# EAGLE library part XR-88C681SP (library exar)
DUAL UART full duplex
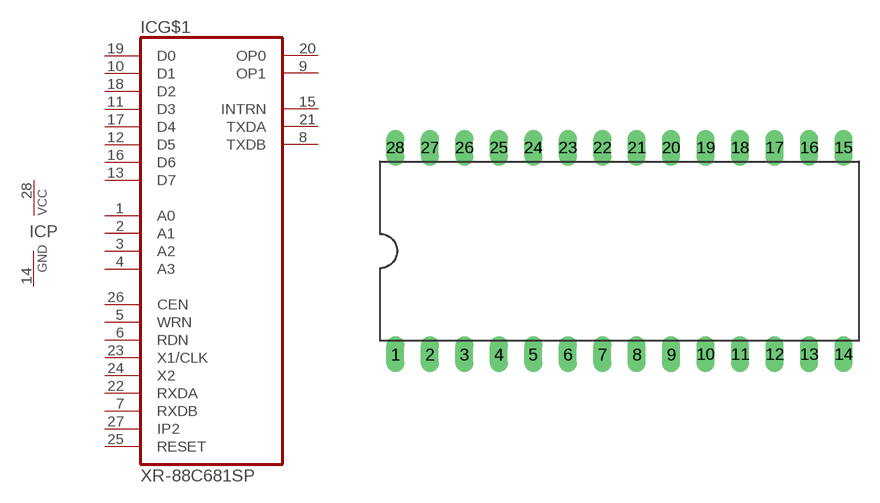
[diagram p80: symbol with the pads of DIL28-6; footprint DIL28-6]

Designator prefix IC; gates G$1=88C681SP P=PWRN

## XR-88C681SP (MPN: XR88C681CP/40-F; OC_FARNELL: 1095818; OC_NEWARK: 53R0425)  [DIL28-6]
1  G$1:A0  in
2  G$1:A1  in
3  G$1:A2  in
4  G$1:A3  in
5  G$1:WRN  in
6  G$1:RDN  in
7  G$1:RXDB  in
8  G$1:TXDB  out
9  G$1:OP1  out
10  G$1:D1
11  G$1:D3
12  G$1:D5
13  G$1:D7
14  P:GND  pwr
15  G$1:INTRN  out
16  G$1:D6
17  G$1:D4
18  G$1:D2
19  G$1:D0
20  G$1:OP0  out
21  G$1:TXDA  out
22  G$1:RXDA  in
23  G$1:X1/CLK  in
24  G$1:X2  in
25  G$1:RESET  in
26  G$1:CEN  in
27  G$1:IP2  in
28  P:VCC  pwr

## Footprint DIL28-6 (pad centres in mm)
Dual In Line Package 0.6 inch
drill 0.813 long: 1 -16.51,-7.62; 2 -13.97,-7.62; 3 -11.43,-7.62; 4 -8.89,-7.62; 5 -6.35,-7.62; 6 -3.81,-7.62; 7 -1.27,-7.62; 8 1.27,-7.62; 9 3.81,-7.62; 10 6.35,-7.62; 11 8.89,-7.62; 12 11.43,-7.62; 13 13.97,-7.62; 14 16.51,-7.62; 15 16.51,7.62; 16 13.97,7.62; 17 11.43,7.62; 18 8.89,7.62; 19 6.35,7.62; 20 3.81,7.62; 21 1.27,7.62; 22 -1.27,7.62; 23 -3.81,7.62; 24 -6.35,7.62; 25 -8.89,7.62; 26 -11.43,7.62; 27 -13.97,7.62; 28 -16.51,7.62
